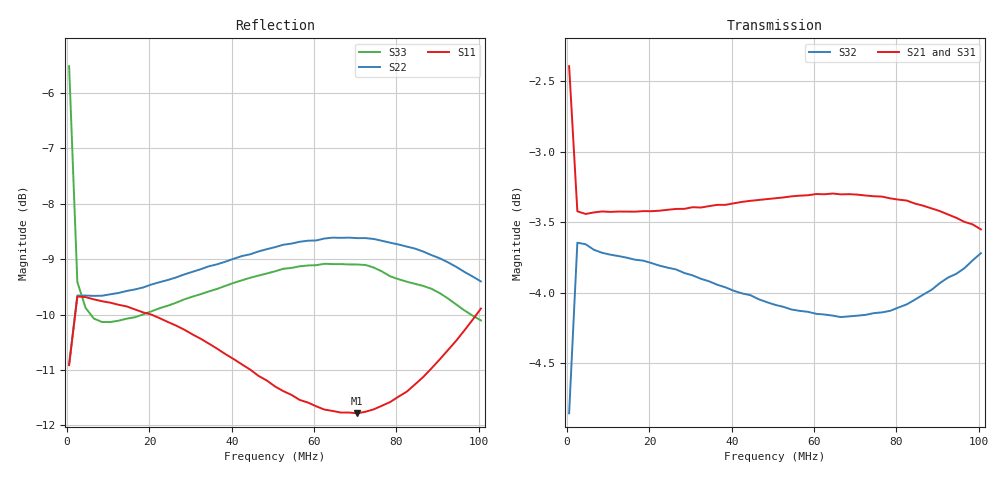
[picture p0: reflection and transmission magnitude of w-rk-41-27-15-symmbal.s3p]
!  Symmetrierer auf Wuerthrinkern OD41mm, ID27mm, H15mm
!  Sat 21/Jul/2018 16:18
#  HZ  s  MA  R 50
!  f [HZ]  S11MAG  S11ANG  S12MAG  S12ANG  S13MAG  S13ANG
!  f [HZ]  S21MAG  S21ANG  S22MAG  S22ANG  S23MAG  S23ANG
!  f [HZ]  S31MAG  S31ANG  S32MAG  S32ANG  S33MAG  S33ANG
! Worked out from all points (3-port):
!   51 points, 500 kHz to 100.5 MHz, reference 50 ohm
!   strongest paths, dB at 500 kHz, 24.5 MHz, 50.5 MHz, 76.5 MHz, 100.5 MHz:
!     S21: -2.4, -3.4, -3.3, -3.3, -3.5
!     S31: -4.9, -3.6, -3.5, -3.5, -3.7
!     S32: -4.9, -3.8, -4.1, -4.1, -3.7
!   lowest |S11| = -11.8 dB at 70.5 MHz (marker M1), VSWR 1.69, Z = 34.1 - j15.2 ohm
!   |S11| at or under -10 dB: start of sweep to 1.971 MHz; 20.5 MHz to 99.41 MHz (78.91 MHz wide, 132 % of centre)
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500000  0.2847 26.8  0.759 -10.5  0.5716 -152.9
        0.7592 -10.5  0.2855 27.6  0.5714 27.5
        0.5715 -152.8  0.5719 27.5  0.5298 88.7
2500000  0.3284 2.4  0.6745 -5.2  0.6581 -176.4
         0.6744 -5.1  0.329 6.3  0.6576 5.5
         0.6578 -176.4  0.6574 5.5  0.3384 24.1
4500000  0.328 -3.6  0.6728 -5.5  0.6577 178.6
         0.673 -5.5  0.329 3.5  0.6567 2.2
         0.6572 178.7  0.6566 2.1  0.3207 12.3
1.05e7  0.3242 -13.8  0.6743 -10.1  0.6541 171.4
        0.6741 -10.0  0.3299 2.4  0.6504 -0.4
        0.6539 171.4  0.651 -0.4  0.3114 5.6
2.85e7  0.3065 -41.7  0.6771 -26.0  0.6602 153.7
        0.6758 -25.8  0.3438 2.1  0.6412 -3.5
        0.6586 153.8  0.6413 -3.4  0.3265 1.8
5.05e7  0.2724 -81.3  0.6837 -46.4  0.6689 131.8
        0.6816 -46.0  0.3638 -0.4  0.6245 -5.2
        0.6666 132.2  0.6249 -5.3  0.346 -3.7
6.05e7  0.2614 -102.8  0.6852 -56.0  0.671 121.6
        0.684 -55.5  0.3689 -2.5  0.6197 -5.4
        0.6697 122.2  0.6203 -5.4  0.3505 -7.1
7.05e7  0.2576 -126.0  0.6843 -65.8  0.6708 111.2
        0.6837 -65.1  0.3707 -5.1  0.6182 -5.4
        0.6704 111.9  0.6194 -5.4  0.3509 -10.9
8.65e7  0.2778 -164.0  0.676 -81.6  0.6618 94.7
        0.6775 -80.7  0.3605 -9.4  0.629 -5.0
        0.6634 95.6  0.6301 -5.0  0.3357 -16.9
1.005e8  0.3202 166.2  0.6607 -95.3  0.6486 80.3
         0.6645 -94.2  0.3388 -12.3  0.6501 -5.4
         0.6529 81.3  0.6518 -5.5  0.3125 -21.6
